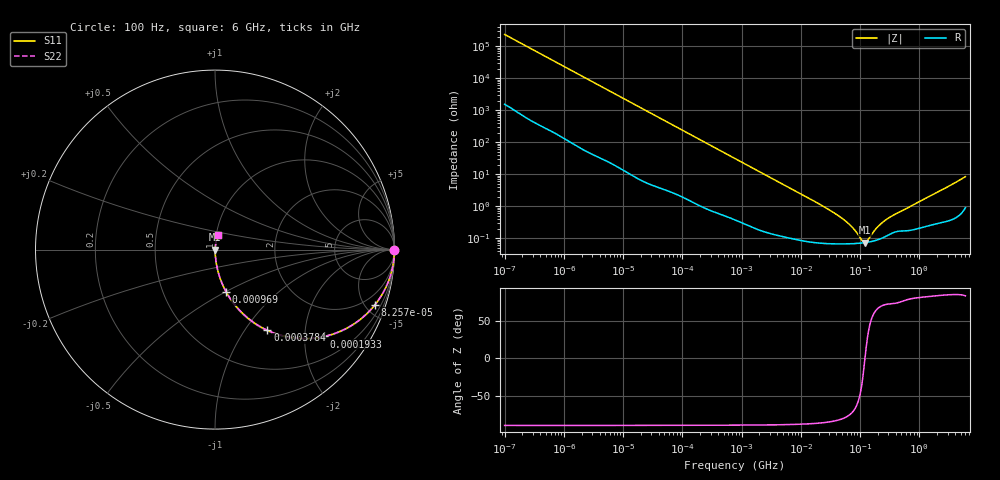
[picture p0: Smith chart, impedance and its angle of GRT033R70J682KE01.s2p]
!Murata Part Number: GRT033R70J682KE01
!These Parameters are Measured in Series Mode Connection
!Data Generated on Jun 19, 2026
!  o--ll--o
!Port1  Port2
!  o------o
!Operation Temp=25[degC], DC Bias Voltage=0[V]
!Freq. Start=100[Hz] Stop=6[GHz] 401[Steps]
# Hz S RI R 50
!Freq.(Hz) S11(Real) S11(Imag) S21(Real) S21(Imag) S12(Real) S12(Imag) S22(Real) S22(Imag)
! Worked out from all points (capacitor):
!   401 points, 100 Hz to 6 GHz, reference 50 ohm
!   read as one part in series: C = 6.78 nF near 109 Hz
!   lowest |Z| = 73.4 mohm at 122 MHz (marker M1)
!   series resonance near 121 MHz, so ESL is about 250 pH
!   S11 on the Smith chart (normalised r, x): 100 Hz: open; 82.57 kHz: 1.05, -5.81; 193.3 kHz: 1.02, -2.49; 378.4 kHz: 1.01, -1.28; 969 kHz: 1.01, -0.50; 6 GHz: 1.02, +0.17
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100  1 -0.000427  3e-06 0.000427  3e-06 0.000427  1 -0.000427
2008  0.9999 -0.00848  0.000116 0.00848  0.000116 0.00848  0.9999 -0.00848
12592  0.9969 -0.0527  0.00307 0.0527  0.00307 0.0527  0.9969 -0.0527
40335  0.9713 -0.1637  0.0287 0.1637  0.0287 0.1637  0.9713 -0.1637
82567  0.8922 -0.3062  0.1078 0.3062  0.1078 0.3062  0.8922 -0.3062
123542  0.7892 -0.4038  0.2108 0.4038  0.2108 0.4038  0.7892 -0.4038
193316  0.6076 -0.4841  0.3924 0.4841  0.3924 0.4841  0.6076 -0.4841
264476  0.4547 -0.4935  0.5453 0.4935  0.5453 0.4935  0.4547 -0.4935
378399  0.2917 -0.4497  0.7083 0.4497  0.7083 0.4497  0.2917 -0.4497
774597  0.0923 -0.2835  0.9077 0.2835  0.9077 0.2835  0.0923 -0.2835
968953  0.0619 -0.2348  0.9381 0.2348  0.9381 0.2348  0.0619 -0.2348
2967816  0.00815 -0.0817  0.9918 0.0817  0.9918 0.0817  0.00815 -0.0817
1.555665e7  0.000991 -0.0156  0.999 0.0156  0.999 0.0156  0.000991 -0.0156
3.330331e7  0.00072 -0.00688  0.9993 0.00688  0.9993 0.00688  0.00072 -0.00688
5.449875e7  0.00068 -0.00363  0.9993 0.00363  0.9993 0.00363  0.00068 -0.00363
7.797396e7  0.000684 -0.00186  0.9993 0.00186  0.9993 0.00186  0.000684 -0.00186
1.115611e8  0.000718 -0.000333  0.9993 0.000333  0.9993 0.000333  0.000718 -0.000333
1.220122e8  0.000733 3.33e-05  0.9993 -3.33e-05  0.9993 -3.33e-05  0.000733 3.33e-05
1.334425e8  0.000751 0.0004  0.9992 -0.0004  0.9992 -0.0004  0.000751 0.0004
1.996653e8  0.000904 0.00211  0.9991 -0.00211  0.9991 -0.00211  0.000904 0.00211
3.124326e8  0.00133 0.00426  0.9987 -0.00426  0.9987 -0.00426  0.00133 0.00426
6e9  0.0158 0.0819  0.9842 -0.0819  0.9842 -0.0819  0.0158 0.0819
